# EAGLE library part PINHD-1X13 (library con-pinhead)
PIN HEADER
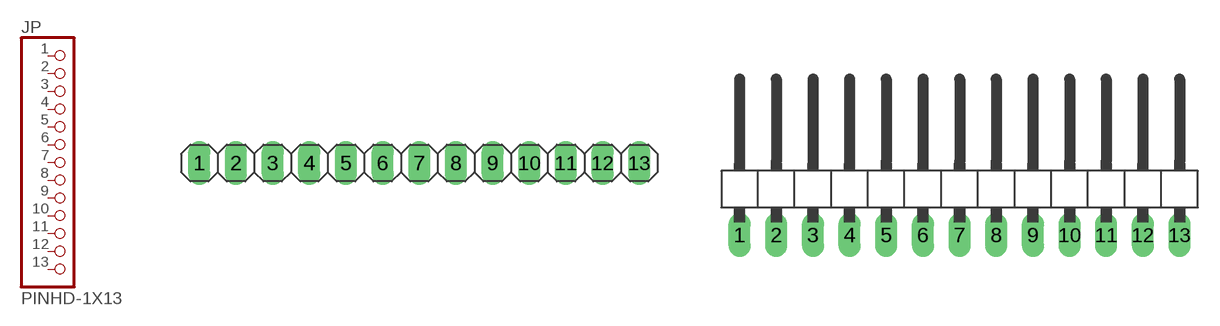
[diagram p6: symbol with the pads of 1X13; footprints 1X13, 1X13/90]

Designator prefix JP

## PINHD-1X13_2.54  [1X13]
1  1  pas
2  2  pas
3  3  pas
4  4  pas
5  5  pas
6  6  pas
7  7  pas
8  8  pas
9  9  pas
10  10  pas
11  11  pas
12  12  pas
13  13  pas

## PINHD-1X13_2.54-90°  [1X13/90]
Pads as for 1X13

## PINHD-1X13_2.00  [1X13M]
Pads as for 1X13

## PINHD-1X13_2.54-SMD  [1X13SMD]
Pads as for 1X13

## PINHD-1X13_2.54-SMD-90°  [1X13SMD/90]
Pads as for 1X13

## Footprint 1X13 (pad centres in mm)
PIN HEADER - 2.54
drill 1.016 long: 1 -15.24,0; 2 -12.7,0; 3 -10.16,0; 4 -7.62,0; 5 -5.08,0; 6 -2.54,0; 7 0,0; 8 2.54,0; 9 5.08,0; 10 7.62,0; 11 10.16,0; 12 12.7,0; 13 15.24,0

## Footprint 1X13/90 (pad centres in mm)
PIN HEADER - 2.54 90°
drill 1.016 long: 1 -15.24,-3.81; 2 -12.7,-3.81; 3 -10.16,-3.81; 4 -7.62,-3.81; 5 -5.08,-3.81; 6 -2.54,-3.81; 7 0,-3.81; 8 2.54,-3.81; 9 5.08,-3.81; 10 7.62,-3.81; 11 10.16,-3.81; 12 12.7,-3.81; 13 15.24,-3.81

## Footprint 1X13M (pad centres in mm)
PIN HEADER - 2
drill 0.914 square: 1 -12,0
drill 0.914: 2 -10,0; 3 -8,0; 4 -6,0; 5 -4,0; 6 -2,0; 7 0,0; 8 2,0; 9 4,0; 10 6,0; 11 8,0; 12 10,0; 13 12,0

## Footprint 1X13SMD (pad centres in mm)
PIN HEADER - 2.54 SMD
smd 1.016 x 3.302: 1 -1.27,1.27; 2 1.27,-1.27; 3 3.81,1.27; 4 6.35,-1.27; 5 8.89,1.27; 6 11.43,-1.27; 7 13.97,1.27; 8 16.51,-1.27; 9 19.05,1.27; 10 21.59,-1.27; 11 24.13,1.27; 12 26.67,-1.27; 13 29.21,1.27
